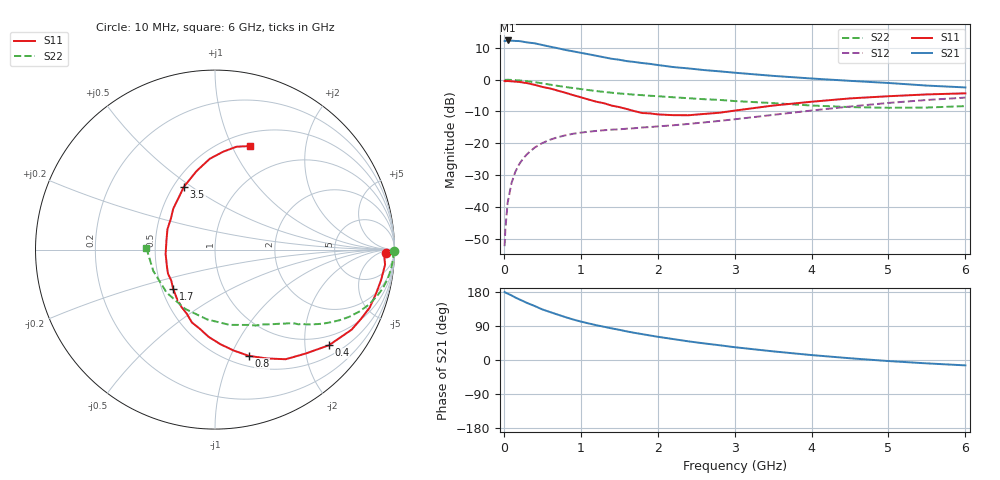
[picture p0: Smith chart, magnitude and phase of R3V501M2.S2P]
! SIEMENS Small Signal Semiconductors
! BFR181
! Si NPN RF Bipolar Junction Transistor in SOT23
! VCE = 0.5 V  IC = 1.2 mA
! Common Emitter S-Parameters:  May  1996
# GHz  S  MA  R  50
!  f  S11  S21  S12  S22
! GHz  MAG  ANG  MAG  ANG  MAG  ANG  MAG  ANG
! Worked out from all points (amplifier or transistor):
!   36 points, 10 MHz to 6 GHz, reference 50 ohm
!   highest |S21| = 12.3 dB at 50 MHz (marker M1)
!   |S21| within 3 dB of that: start of sweep to 803.4 MHz
!   unconditionally stable (mu >= 1): 1.683 GHz to 4.341 GHz
!   at 250 MHz: K = 0.19, MSG = 18.4 dB, |S12| = -24.8 dB
!   at 1.4 GHz: K = 0.88, MSG = 11.2 dB, |S12| = -15.7 dB
!   at 6 GHz: K = 0.97, MSG = 1.6 dB, |S12| = -5.6 dB
!   S11 on the Smith chart (normalised r, x): 10 MHz: 35, -14; 400 MHz: 0.75, -2.55; 800 MHz: 0.61, -1.17; 1.7 GHz: 0.57, -0.28; 3.5 GHz: 0.57, +0.47; 6 GHz: 0.64, +1.17
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0.01  0.9516 -1.1  4.063 179.4  0.0024 87.4  0.9967 -0.5
0.02  0.9435 -2.0  4.027 178.0  0.0045 88.6  0.9909 -1.1
0.05  0.9512 -5.1  4.133 175.2  0.0117 85.9  0.9947 -2.7
0.1  0.9408 -10.4  4.102 170.5  0.0237 84.0  0.9888 -5.3
0.15  0.9298 -15.5  4.06 164.8  0.0356 79.9  0.9812 -8.0
0.2  0.9203 -20.6  4.042 160.1  0.0468 77.0  0.9719 -10.4
0.3  0.882 -30.4  3.853 150.7  0.067 70.8  0.9438 -15.3
0.4  0.8289 -40.0  3.729 142.5  0.0853 65.2  0.9128 -19.5
0.5  0.7685 -48.9  3.508 133.5  0.1005 60.4  0.8743 -23.3
0.6  0.7267 -57.2  3.302 126.6  0.1134 56.0  0.8352 -26.7
0.8  0.6216 -72.3  2.931 113.2  0.1329 49.4  0.7662 -31.8
0.9  0.5713 -79.6  2.787 106.9  0.1408 46.8  0.738 -33.8
1.1  0.4868 -94.3  2.509 96.6  0.1518 43.0  0.6854 -37.4
1.4  0.3907 -113.7  2.131 83.5  0.1632 39.8  0.623 -41.9
1.7  0.3192 -137.0  1.895 71.6  0.1721 39.0  0.5795 -45.1
1.9  0.2944 -152.8  1.77 64.7  0.1794 39.2  0.5575 -47.7
2.2  0.2762 -174.8  1.578 55.3  0.1913 40.0  0.5283 -51.8
2.8  0.301 144.6  1.352 39.0  0.2242 42.0  0.4802 -61.8
3.5  0.391 116.2  1.146 22.8  0.279 41.6  0.4273 -79.0
4.5  0.5068 93.3  0.957 4.6  0.3776 35.3  0.3698 -116.7
5.5  0.5856 78.2  0.806 -8.9  0.4787 23.7  0.3638 -160.9
6  0.6088 71.4  0.754 -14.2  0.5218 16.7  0.3835 178.3
